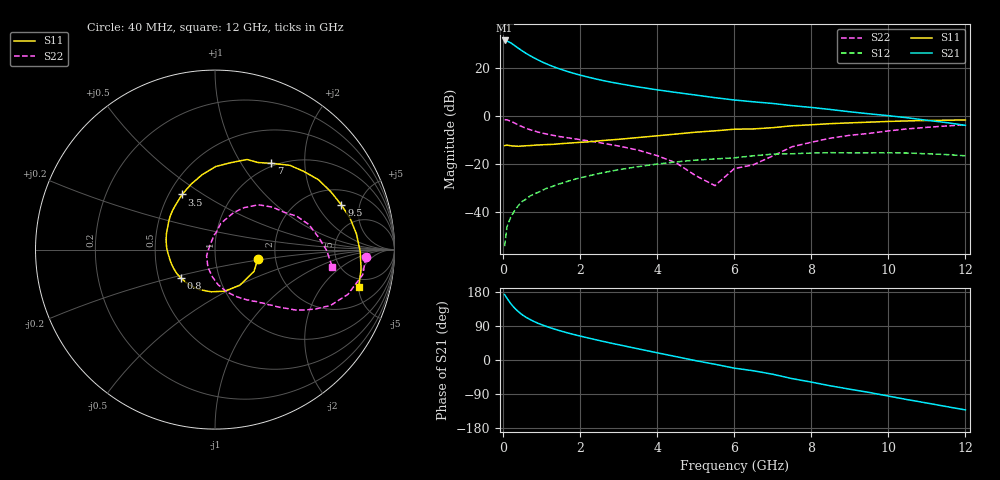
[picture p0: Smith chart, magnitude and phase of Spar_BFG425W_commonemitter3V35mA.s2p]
! Filename: 335bfg425.001
! BFG425W Field C1
! V1=8.585E-001V,V2=3.000E+000V, I1=5.159E-004A, I2=3.507E-002A
# GHz  S  MA  R 50
!  S11  S21  S12  S22
!Freq(GHz)  Mag  Ang  Mag  Ang  Mag  Ang  Mag  Ang
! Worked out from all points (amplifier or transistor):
!   44 points, 40 MHz to 12 GHz, reference 50 ohm
!   highest |S21| = 31.4 dB at 40 MHz (marker M1)
!   |S21| within 3 dB of that: start of sweep to 376.8 MHz
!   unconditionally stable (mu >= 1): start of sweep to 84.11 MHz; 818.9 MHz to end of sweep
!   at 700 MHz: K = 0.95, MSG = 29.1 dB, |S12| = -33.2 dB
!   at 2.4 GHz: K = 1.24, MAG = 16.8 dB, |S12| = -24.2 dB
!   at 12 GHz: K = 1.40, MAG = 2.6 dB, |S12| = -16.5 dB
!   S11 on the Smith chart (normalised r, x): 40 MHz: 1.61, -0.18; 800 MHz: 0.65, -0.22; 3.5 GHz: 0.58, +0.41; 7 GHz: 0.96, +1.37; 9.5 GHz: 2.96, +3.33; 12 GHz: 3.83, -5.04
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0.04  0.244 -12.6  36.97 172.7  0.002 59.9  0.842 -3.0
0.1  0.249 -29.2  36.09 163.2  0.005 75.7  0.835 -9.6
0.2  0.242 -55.3  33 148.6  0.008 71.8  0.781 -18.6
0.3  0.238 -76.9  28.96 136.9  0.011 68.9  0.715 -25.8
0.4  0.236 -95.2  25.38 127.3  0.014 67.2  0.65 -30.6
0.5  0.239 -110.7  22.39 119.1  0.017 65.0  0.601 -34.1
0.6  0.242 -122.4  19.89 112.5  0.019 64.1  0.557 -37.1
0.8  0.248 -140.6  16.15 101.8  0.024 62.5  0.493 -41.1
1  0.253 -155.0  13.42 93.2  0.028 61.3  0.446 -44.1
1.3  0.259 -171.2  10.63 82.7  0.035 59.3  0.398 -48.4
1.7  0.274 172.2  8.272 70.8  0.045 56.1  0.352 -54.3
2.2  0.291 155.3  6.437 58.4  0.057 50.7  0.307 -61.8
2.8  0.32 138.1  5.051 44.6  0.072 43.2  0.255 -71.8
3.5  0.358 120.8  4.025 29.6  0.089 33.5  0.197 -84.8
4.5  0.424 99.6  3.078 8.7  0.112 18.4  0.106 -111.8
5.5  0.493 79.5  2.406 -11.3  0.129 2.7  0.036 147.6
6.5  0.541 63.7  1.975 -28.4  0.15 -9.8  0.098 85.4
7  0.574 56.8  1.824 -37.6  0.162 -17.5  0.149 77.6
8.5  0.696 34.0  1.367 -68.2  0.174 -46.2  0.348 45.9
9.5  0.747 19.4  1.113 -85.5  0.172 -62.5  0.437 28.4
10.5  0.793 6.3  0.92 -104.7  0.171 -80.7  0.542 14.8
12  0.828 -14.5  0.641 -131.7  0.15 -109.9  0.66 -8.3
